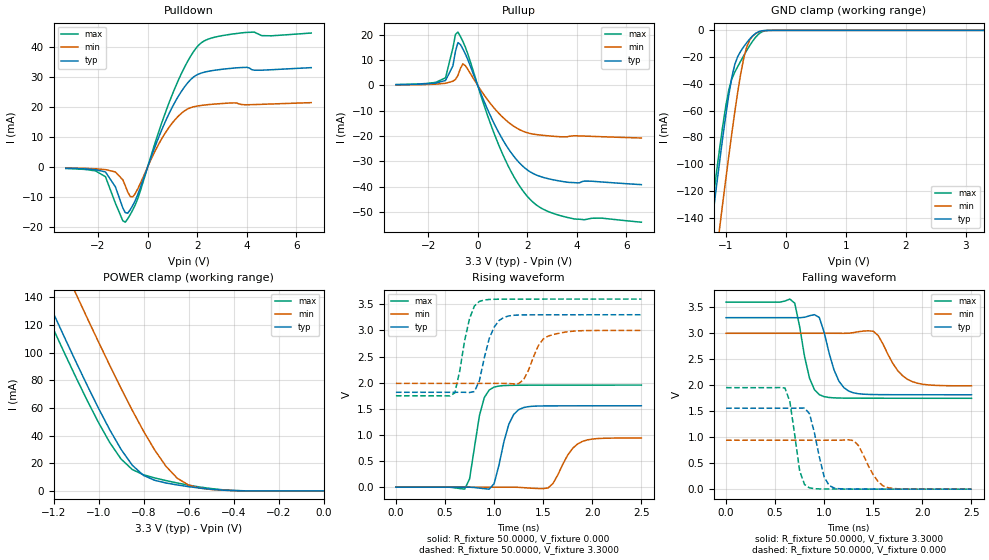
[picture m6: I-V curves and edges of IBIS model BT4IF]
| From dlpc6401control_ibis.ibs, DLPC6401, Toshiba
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[Model]   BT4IF
Model_type   3-state
Polarity   Non-Inverting
Enable   Active-Low
C_comp   1.414pF   NA   NA
Vmeas = 1.40V
|Variable   typ   min   max
[Voltage range]  3.3   3.0   3.6
[Temperature Range]   25.0000   125.000   0.000
[Pullup Reference]   3.3000V   3.0000V   3.6000V
[Pulldown Reference]   0.000V   0.000V   0.000V
[POWER Clamp Reference]   3.3000V   3.0000V   3.6000V
[GND Clamp Reference]   0.000V   0.000V   0.000V
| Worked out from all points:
|   slope of the pulldown table from 0 to 0.495 V, typ, clamps not added: 45.5 ohm
|   slope of the pullup table from 0 to 0.495 V, typ, clamps not added: 42.6 ohm
|   GND clamp passes 1 mA (typ) near -0.45 V on its own axis
|   POWER clamp passes 1 mA (typ) near -0.48 V on its own axis
|   rising waveform, R_fixture 50.0000, V_fixture 0.000: 20-80 % time 127ps typ, 171ps min, 109ps max; typ from 0 V to 1.56 V
|   rising waveform, R_fixture 50.0000, V_fixture 3.3000: 20-80 % time 128ps typ, 149ps min, 113ps max; typ from 1.82 V to 3.3 V
|   falling waveform, R_fixture 50.0000, V_fixture 3.3000: 20-80 % time 140ps typ, 197ps min, 116ps max; typ from 3.3 V to 1.82 V
|   falling waveform, R_fixture 50.0000, V_fixture 0.000: 20-80 % time 112ps typ, 160ps min, 87.5ps max; typ from 1.56 V to 0 V
[Pulldown]
| voltage   I(typ)   I(min)   I(max)
-3.3V     -367.7uA   -282.2uA   -461.6uA
-1.7V     -1.6mA     -833.4uA   -3.189mA
-1.3V     -6.539mA   -1.61mA    -11.98mA
-900mV    -15.15mA   -6.21mA    -18.3mA
-600mV    -12.75mA   -9.885mA   -14.26mA
-300mV    -6.971mA   -5.535mA   -8.073mA
400mV     8.942mA    6.898mA    10.53mA
950mV     19.18mA    14.16mA    23.16mA
1.55V     27.3mA     19mA       34.13mA
2.05V     30.88mA    20.35mA    40.42mA
3.9V      33.11mA    20.72mA    44.68mA
6.6V      33.04mA    21.41mA    44.53mA
[Pullup]
| voltage   I(typ)   I(min)   I(max)
-3.3V     291.2uA    192.2uA    349.5uA
-1.3V     1.955mA    843.2uA    2.989mA
-1V       7.776mA    1.666mA    14.86mA
-900mV    13.41mA    2.394mA    20.14mA
-800mV    16.9mA     3.889mA    21.06mA
-600mV    14.43mA    8.546mA    17.37mA
-500mV    12.45mA    7.801mA    15.09mA
950mV     -20.41mA   -12mA      -25.89mA
1.55V     -29.11mA   -16.7mA    -37.57mA
2.1V      -34.02mA   -18.94mA   -44.86mA
3.8V      -38.34mA   -19.93mA   -52.52mA
6.6V      -39.16mA   -20.75mA   -53.99mA
[GND_clamp]
| voltage   I(typ)   I(min)   I(max)
-3.3V     -944.9mA   -993.5mA   -933.7mA
-1.3V     -169.6mA   -220.5mA   -158.5mA
-1.25V    -151.2mA   -201.9mA   -140.2mA
-1.2V     -132.9mA   -183.4mA   -122.2mA
-1.1V     -97.21mA   -147mA     -87.47mA
-1V       -63.63mA   -111.4mA   -56.62mA
-900mV    -35.29mA   -77.26mA   -36.39mA
-800mV    -19.53mA   -45.93mA   -27.04mA
-700mV    -12.2mA    -20.73mA   -18.85mA
-600mV    -6.422mA   -7.153mA   -11.28mA
-450mV    -954.9uA   -1.183mA   -2.691mA
3.3V      2.12nA     24.26uA    12.22nA
[POWER_clamp]
| voltage   I(typ)   I(min)   I(max)
-3.3V     917.5mA    964.8mA    906.4mA
-1.3V     164.1mA    213.9mA    152.5mA
-1.25V    146mA      195.8mA    134.5mA
-1.2V     128.2mA    177.9mA    116.7mA
-1.1V     93.14mA    142.3mA    81.92mA
-950mV    44.15mA    90.68mA    34.95mA
-850mV    18.58mA    58.26mA    15.44mA
-750mV    7.652mA    29.46mA    9.374mA
-650mV    4.312mA    9.163mA    5.736mA
-600mV    3.088mA    4.252mA    4.184mA
-500mV    1.206mA    1.062mA    1.712mA
0V        2.118nA    56.3nA     15.39nA
[Ramp]
| variable   typ   min   max
dV/dt_r   0.9348/0.1197n   0.5647/0.1660n   1.1723/99.1520p
dV/dt_f   0.8900/0.1366n   0.6071/0.1955n   1.1106/0.1104n
R_load = 50.0000
[Rising Waveform]
R_fixture = 50.0000
V_fixture = 0.000
V_fixture_min = 0.000
V_fixture_max = 0.000
| time   V(typ)   V(min)   V(max)
0s        0V         0V         0V
700ps     190.8uV    5.207uV    -36.91mV
750ps     77.38uV    2.643uV    157.3mV
900ps     -28.44mV   -5.995uV   1.715V
1ns       66.5mV     -2.637uV   1.915V
1.15ns    1.205V     350.2uV    1.948V
1.25ns    1.483V     -2.747mV   1.951V
1.55ns    1.556V     -13.16mV   1.953V
1.9ns     1.557V     876.4mV    1.953V
2.5ns     1.558V     941.2mV    1.954V
[Rising Waveform]
R_fixture = 50.0000
V_fixture = 3.3000
V_fixture_min = 3.0000
V_fixture_max = 3.6000
| time   V(typ)   V(min)   V(max)
0s        1.816V     1.987V     1.749V
600ps     1.816V     1.987V     1.805V
750ps     1.812V     1.987V     3.228V
850ps     2.036V     1.987V     3.555V
950ps     2.843V     1.987V     3.592V
1.1ns     3.249V     1.986V     3.598V
1.3ns     3.297V     2.055V     3.599V
1.45ns    3.299V     2.706V     3.599V
1.55ns    3.299V     2.891V     3.599V
2.5ns     3.3V       3V         3.6V
[Falling Waveform]
R_fixture = 50.0000
V_fixture = 3.3000
V_fixture_min = 3.0000
V_fixture_max = 3.6000
| time   V(typ)   V(min)   V(max)
0s        3.3V       3V         3.6V
700ps     3.3V       3V         3.578V
850ps     3.338V     3V         2.138V
950ps     3.303V     3V         1.819V
1ns       3.014V     3V         1.78V
1.1ns     2.294V     3V         1.757V
1.25ns    1.887V     3.001V     1.752V
1.5ns     1.821V     3.038V     1.75V
1.9ns     1.817V     2.067V     1.749V
2.5ns     1.817V     1.988V     1.749V
[Falling Waveform]
R_fixture = 50.0000
V_fixture = 0.000
V_fixture_min = 0.000
V_fixture_max = 0.000
| time   V(typ)   V(min)   V(max)
0s        1.558V     941.9mV    1.954V
600ps     1.558V     942mV      1.947V
650ps     1.558V     942mV      1.687V
750ps     1.56V      942mV      350mV
850ps     1.453V     942mV      24.53mV
1ns       232.5mV    941.9mV    3.516mV
1.1ns     22.86mV    941.6mV    2.45mV
1.3ns     2.169mV    933.2mV    1.377mV
1.65ns    858.8uV    28.56mV    507.4uV
2.5ns     139.9uV    318.7uV    85.38uV
